FUNCTION "CONSENSI" : VOID
TITLE =CONSENSI
VERSION : 0.1

BEGIN
NETWORK
TITLE =CONS AV FLUSSAGGIO
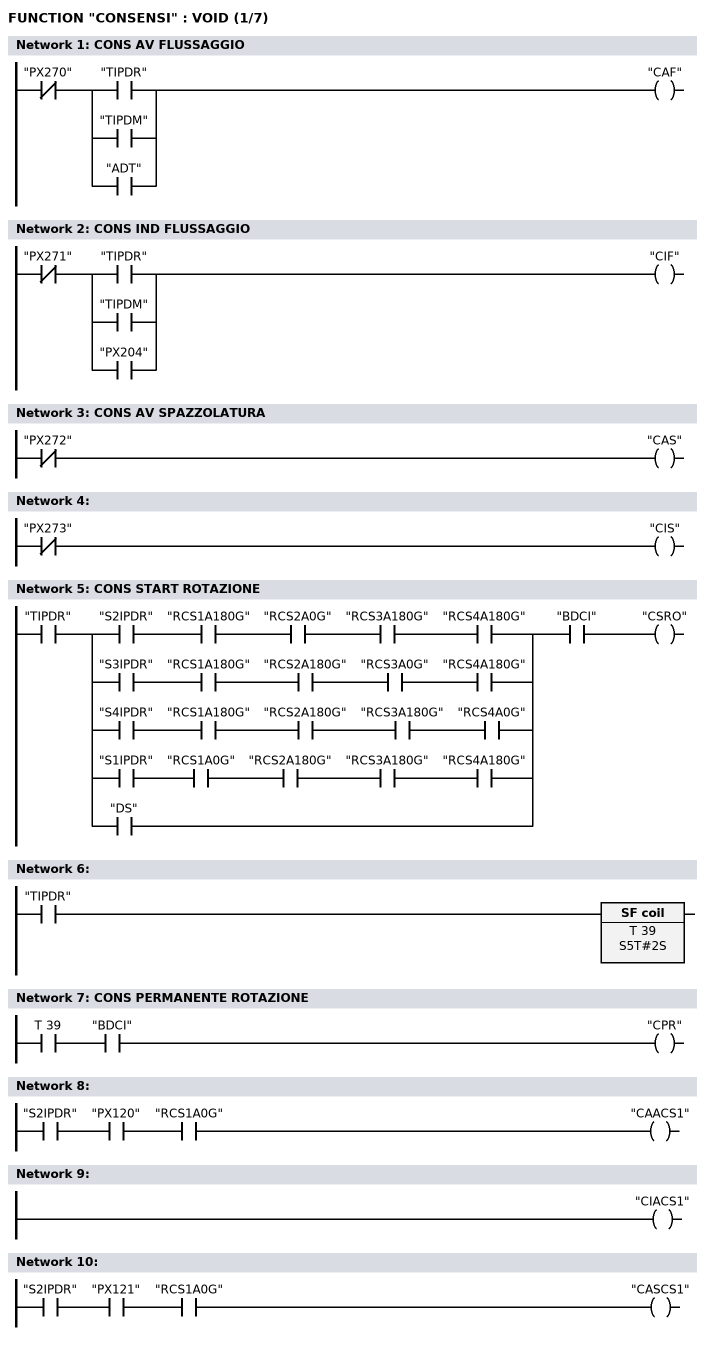
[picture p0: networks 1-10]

      UN    "PX270";
      U(    ;
      O     "TIPDR";
      O     "TIPDM";
      O     "ADT";
      )     ;
      =     "CAF";
NETWORK
TITLE =CONS IND FLUSSAGGIO

      UN    "PX271";
      U(    ;
      O     "TIPDR";
      O     "TIPDM";
      O     "PX204";
      )     ;
      =     "CIF";
NETWORK
TITLE =CONS AV SPAZZOLATURA

      UN    "PX272";
      =     "CAS";
NETWORK
TITLE =

      UN    "PX273";
      =     "CIS";
NETWORK
TITLE =CONS START ROTAZIONE

      U     "TIPDR";
      U(    ;
      U     "S2IPDR";
      U     "RCS1A180G";
      U     "RCS2A0G";
      U     "RCS3A180G";
      U     "RCS4A180G";
      O     ;
      U     "S3IPDR";
      U     "RCS1A180G";
      U     "RCS2A180G";
      U     "RCS3A0G";
      U     "RCS4A180G";
      O     ;
      U     "S4IPDR";
      U     "RCS1A180G";
      U     "RCS2A180G";
      U     "RCS3A180G";
      U     "RCS4A0G";
      O     ;
      U     "S1IPDR";
      U     "RCS1A0G";
      U     "RCS2A180G";
      U     "RCS3A180G";
      U     "RCS4A180G";
      O     "DS";
      )     ;
      U     "BDCI";
      =     "CSRO";
NETWORK
TITLE =

      U     "TIPDR";
      L     S5T#2S;
      SA    T     39;
NETWORK
TITLE =CONS PERMANENTE ROTAZIONE

      U     T     39;
      U     "BDCI";
      =     "CPR";
NETWORK
TITLE =

      U     "S2IPDR";
      U     "PX120";
      U     "RCS1A0G";
      =     "CAACS1";
NETWORK
TITLE =

      SET   ;
      =     "CIACS1";
NETWORK
TITLE =

      U     "S2IPDR";
      U     "PX121";
      U     "RCS1A0G";
      =     "CASCS1";
NETWORK
TITLE =
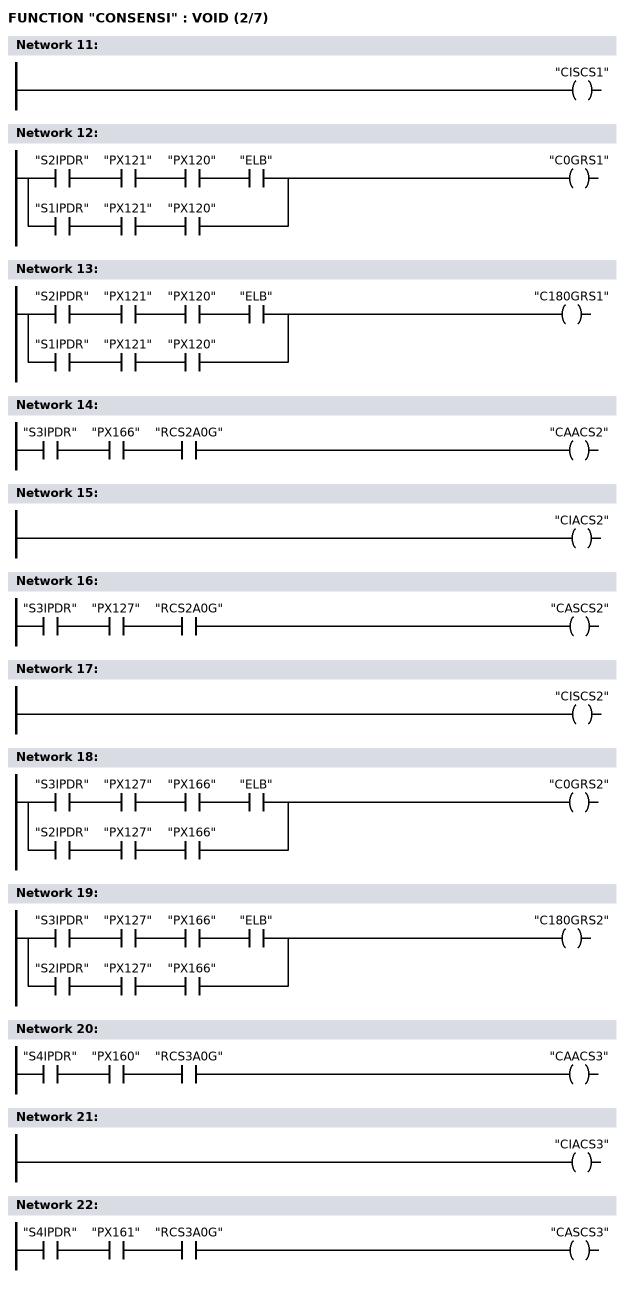
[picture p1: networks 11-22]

      SET   ;
      =     "CISCS1";
NETWORK
TITLE =

      U     "S2IPDR";
      U     "PX121";
      U     "PX120";
      U     "ELB";
      O     ;
      U     "S1IPDR";
      U     "PX121";
      U     "PX120";
      =     "C0GRS1";
NETWORK
TITLE =

      U     "S2IPDR";
      U     "PX121";
      U     "PX120";
      U     "ELB";
      O     ;
      U     "S1IPDR";
      U     "PX121";
      U     "PX120";
      =     "C180GRS1";
NETWORK
TITLE =

      U     "S3IPDR";
      U     "PX166";
      U     "RCS2A0G";
      =     "CAACS2";
NETWORK
TITLE =

      SET   ;
      =     "CIACS2";
NETWORK
TITLE =

      U     "S3IPDR";
      U     "PX127";
      U     "RCS2A0G";
      =     "CASCS2";
NETWORK
TITLE =

      SET   ;
      =     "CISCS2";
NETWORK
TITLE =

      U     "S3IPDR";
      U     "PX127";
      U     "PX166";
      U     "ELB";
      O     ;
      U     "S2IPDR";
      U     "PX127";
      U     "PX166";
      =     "C0GRS2";
NETWORK
TITLE =

      U     "S3IPDR";
      U     "PX127";
      U     "PX166";
      U     "ELB";
      O     ;
      U     "S2IPDR";
      U     "PX127";
      U     "PX166";
      =     "C180GRS2";
NETWORK
TITLE =

      U     "S4IPDR";
      U     "PX160";
      U     "RCS3A0G";
      =     "CAACS3";
NETWORK
TITLE =

      SET   ;
      =     "CIACS3";
NETWORK
TITLE =

      U     "S4IPDR";
      U     "PX161";
      U     "RCS3A0G";
      =     "CASCS3";
NETWORK
TITLE =
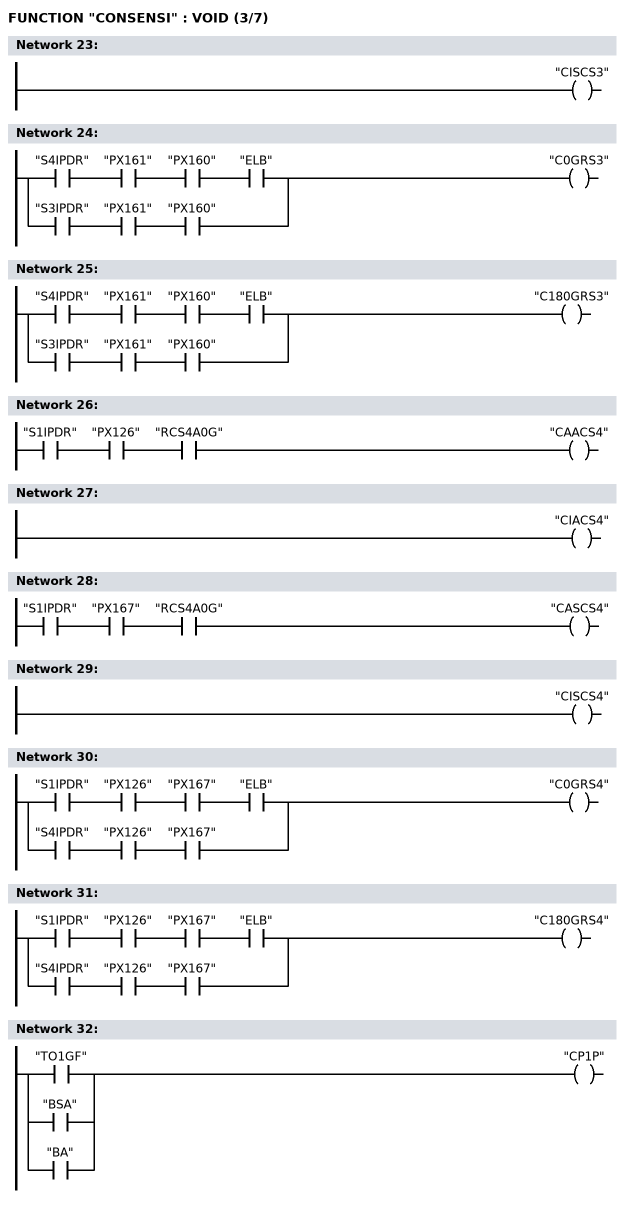
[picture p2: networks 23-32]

      SET   ;
      =     "CISCS3";
NETWORK
TITLE =

      U     "S4IPDR";
      U     "PX161";
      U     "PX160";
      U     "ELB";
      O     ;
      U     "S3IPDR";
      U     "PX161";
      U     "PX160";
      =     "C0GRS3";
NETWORK
TITLE =

      U     "S4IPDR";
      U     "PX161";
      U     "PX160";
      U     "ELB";
      O     ;
      U     "S3IPDR";
      U     "PX161";
      U     "PX160";
      =     "C180GRS3";
NETWORK
TITLE =

      U     "S1IPDR";
      U     "PX126";
      U     "RCS4A0G";
      =     "CAACS4";
NETWORK
TITLE =

      SET   ;
      =     "CIACS4";
NETWORK
TITLE =

      U     "S1IPDR";
      U     "PX167";
      U     "RCS4A0G";
      =     "CASCS4";
NETWORK
TITLE =

      SET   ;
      =     "CISCS4";
NETWORK
TITLE =

      U     "S1IPDR";
      U     "PX126";
      U     "PX167";
      U     "ELB";
      O     ;
      U     "S4IPDR";
      U     "PX126";
      U     "PX167";
      =     "C0GRS4";
NETWORK
TITLE =

      U     "S1IPDR";
      U     "PX126";
      U     "PX167";
      U     "ELB";
      O     ;
      U     "S4IPDR";
      U     "PX126";
      U     "PX167";
      =     "C180GRS4";
NETWORK
TITLE =

      O     "TO1GF";
      O     "BSA";
      O     "BA";
      =     "CP1P";
NETWORK
TITLE =
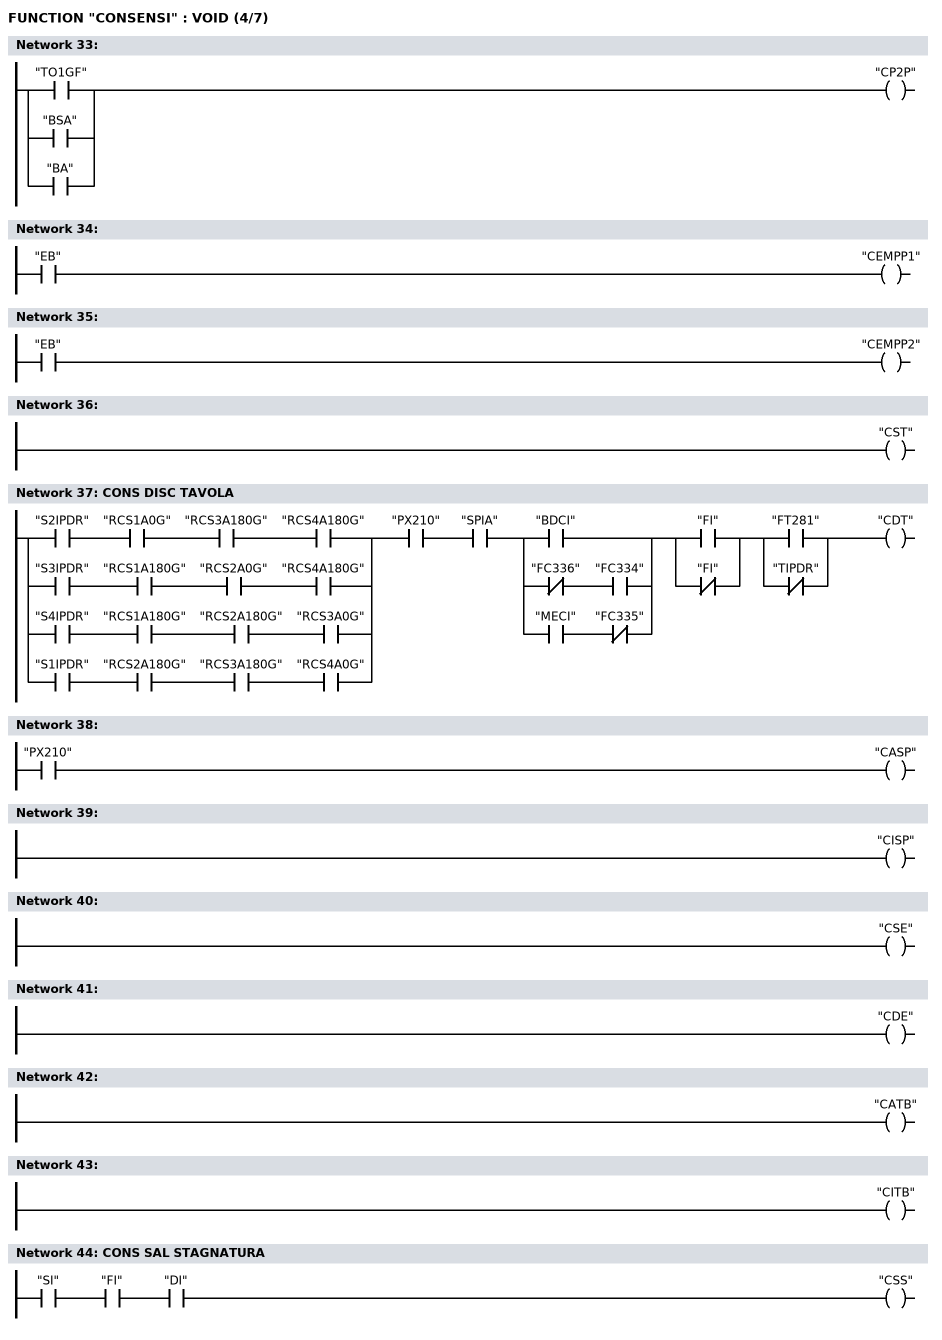
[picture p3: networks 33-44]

      O     "TO1GF";
      O     "BSA";
      O     "BA";
      =     "CP2P";
NETWORK
TITLE =

      U     "EB";
      =     "CEMPP1";
NETWORK
TITLE =

      U     "EB";
      =     "CEMPP2";
NETWORK
TITLE =

      SET   ;
      =     "CST";
NETWORK
TITLE =CONS DISC TAVOLA

      U(    ;
      U     "S2IPDR";
      U     "RCS1A0G";
      U     "RCS3A180G";
      U     "RCS4A180G";
      O     ;
      U     "S3IPDR";
      U     "RCS1A180G";
      U     "RCS2A0G";
      U     "RCS4A180G";
      O     ;
      U     "S4IPDR";
      U     "RCS1A180G";
      U     "RCS2A180G";
      U     "RCS3A0G";
      O     ;
      U     "S1IPDR";
      U     "RCS2A180G";
      U     "RCS3A180G";
      U     "RCS4A0G";
      )     ;
      U     "PX210";
      U     "SPIA";
      U(    ;
      O     "BDCI";
      O     ;
      UN    "FC336";
      U     "FC334";
      O     ;
      U     "MECI";
      UN    "FC335";
      )     ;
      U(    ;
      O     "FI";
      ON    "FI";
      )     ;
      U(    ;
      O     "FT281";
      ON    "TIPDR";
      )     ;
      =     "CDT";
NETWORK
TITLE =

      U     "PX210";
      =     "CASP";
NETWORK
TITLE =

      SET   ;
      =     "CISP";
NETWORK
TITLE =

      SET   ;
      =     "CSE";
NETWORK
TITLE =

      SET   ;
      =     "CDE";
NETWORK
TITLE =

      SET   ;
      =     "CATB";
NETWORK
TITLE =

      SET   ;
      =     "CITB";
NETWORK
TITLE =CONS SAL STAGNATURA

      U     "SI";
      U     "FI";
      U     "DI";
      =     "CSS";
NETWORK
TITLE =
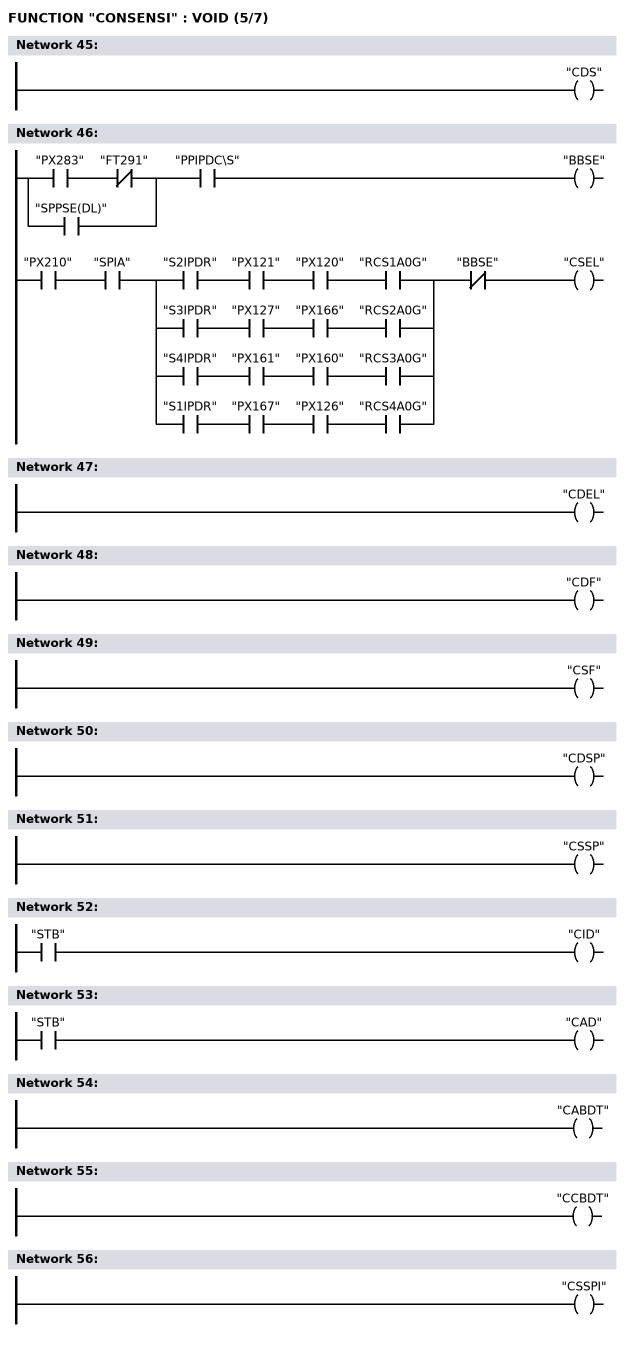
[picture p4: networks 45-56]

      SET   ;
      =     "CDS";
NETWORK
TITLE =

      U(    ;
      U     "PX283";
      UN    "FT291";
      O     ;
      U     "SPPSE(DL)";
      )     ;
      U     "PPIPDC\S";
      =     "BBSE";
      U     "PX210";
      U     "SPIA";
      U(    ;
      U     "S2IPDR";
      U     "PX121";
      U     "PX120";
      U     "RCS1A0G";
      O     ;
      U     "S3IPDR";
      U     "PX127";
      U     "PX166";
      U     "RCS2A0G";
      O     ;
      U     "S4IPDR";
      U     "PX161";
      U     "PX160";
      U     "RCS3A0G";
      O     ;
      U     "S1IPDR";
      U     "PX167";
      U     "PX126";
      U     "RCS4A0G";
      )     ;
      UN    "BBSE";
      =     "CSEL";
NETWORK
TITLE =

      SET   ;
      =     "CDEL";
NETWORK
TITLE =

      SET   ;
      =     "CDF";
NETWORK
TITLE =

      SET   ;
      =     "CSF";
NETWORK
TITLE =

      SET   ;
      =     "CDSP";
NETWORK
TITLE =

      SET   ;
      =     "CSSP";
NETWORK
TITLE =

      U     "STB";
      =     "CID";
NETWORK
TITLE =

      U     "STB";
      =     "CAD";
NETWORK
TITLE =

      SET   ;
      =     "CABDT";
NETWORK
TITLE =

      SET   ;
      =     "CCBDT";
NETWORK
TITLE =

      SET   ;
      =     "CSSPI";
NETWORK
TITLE =
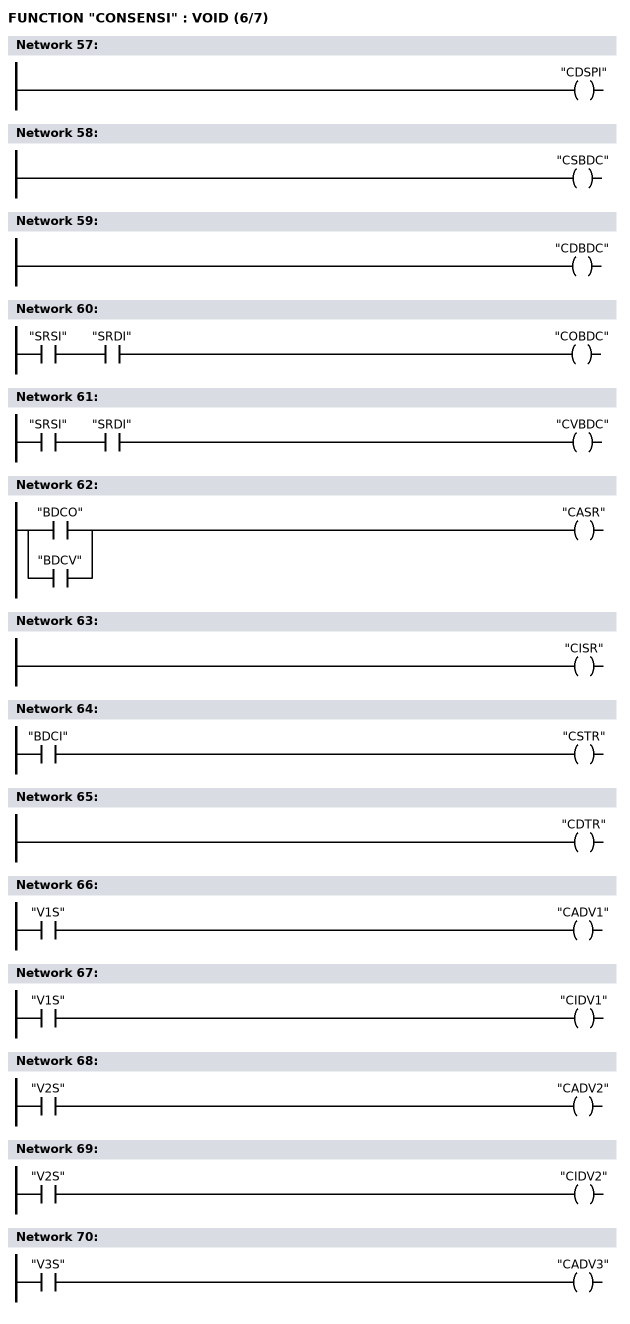
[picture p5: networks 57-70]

      SET   ;
      =     "CDSPI";
NETWORK
TITLE =

      SET   ;
      =     "CSBDC";
NETWORK
TITLE =

      SET   ;
      =     "CDBDC";
NETWORK
TITLE =

      U     "SRSI";
      U     "SRDI";
      =     "COBDC";
NETWORK
TITLE =

      U     "SRSI";
      U     "SRDI";
      =     "CVBDC";
NETWORK
TITLE =

      O     "BDCO";
      O     "BDCV";
      =     "CASR";
NETWORK
TITLE =

      SET   ;
      =     "CISR";
NETWORK
TITLE =

      U     "BDCI";
      =     "CSTR";
NETWORK
TITLE =

      SET   ;
      =     "CDTR";
NETWORK
TITLE =

      U     "V1S";
      =     "CADV1";
NETWORK
TITLE =

      U     "V1S";
      =     "CIDV1";
NETWORK
TITLE =

      U     "V2S";
      =     "CADV2";
NETWORK
TITLE =

      U     "V2S";
      =     "CIDV2";
NETWORK
TITLE =

      U     "V3S";
      =     "CADV3";
NETWORK
TITLE =
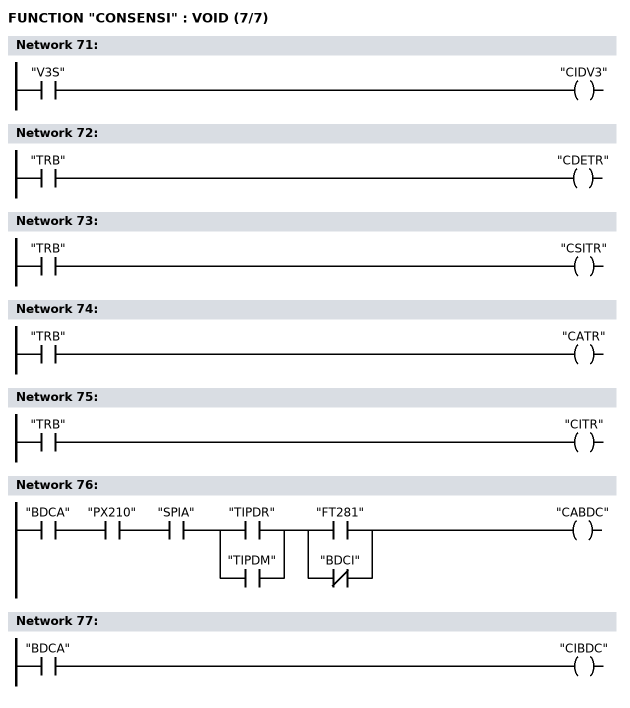
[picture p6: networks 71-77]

      U     "V3S";
      =     "CIDV3";
NETWORK
TITLE =

      U     "TRB";
      =     "CDETR";
NETWORK
TITLE =

      U     "TRB";
      =     "CSITR";
NETWORK
TITLE =

      U     "TRB";
      =     "CATR";
NETWORK
TITLE =

      U     "TRB";
      =     "CITR";
NETWORK
TITLE =

      U     "BDCA";
      U     "PX210";
      U     "SPIA";
      U(    ;
      O     "TIPDR";
      O     "TIPDM";
      )     ;
      U(    ;
      O     "FT281";
      ON    "BDCI";
      )     ;
      =     "CABDC";
NETWORK
TITLE =

      U     "BDCA";
      =     "CIBDC";
END_FUNCTION

